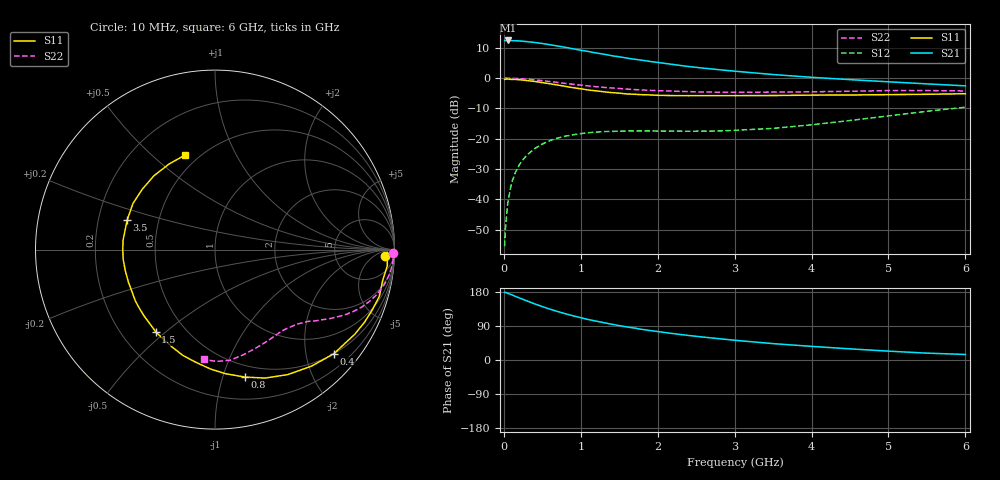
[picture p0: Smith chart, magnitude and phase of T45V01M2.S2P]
! Infineon Technologies  Discrete & RF Semiconductors
! BFR182T
! Si NPN RF Bipolar Junction Transistor in SC75
! VCE = 5 V  IC = 1.2 mA
! Common Emitter S-Parameters:  October  1999
# GHz  S  MA  R  50
!  f  S11  S21  S12  S22
! GHz  MAG  ANG  MAG  ANG  MAG  ANG  MAG  ANG
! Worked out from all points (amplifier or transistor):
!   36 points, 10 MHz to 6 GHz, reference 50 ohm
!   highest |S21| = 12.4 dB at 50 MHz (marker M1)
!   |S21| within 3 dB of that: start of sweep to 950.9 MHz
!   unconditionally stable (mu >= 1): 2.324 GHz to 4.534 GHz
!   at 250 MHz: K = 0.11, MSG = 19.5 dB, |S12| = -26.9 dB
!   at 1.4 GHz: K = 0.62, MSG = 12.5 dB, |S12| = -17.6 dB
!   at 6 GHz: K = 0.83, MSG = 3.5 dB, |S12| = -9.6 dB
!   S11 on the Smith chart (normalised r, x): 10 MHz: 25, -19; 400 MHz: 0.50, -2.58; 800 MHz: 0.39, -1.19; 1.5 GHz: 0.34, -0.46; 3.5 GHz: 0.33, +0.15; 6 GHz: 0.42, +0.64
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0.01  0.9503 -2.2  4.144 178.6  0.0017 80.0  0.9902 -1.1
0.02  0.96 -0.8  4.134 178.7  0.0032 92.0  0.9999 -0.9
0.05  0.9644 -5.4  4.171 176.0  0.0086 89.7  0.9971 -2.1
0.1  0.9502 -10.2  4.132 172.3  0.0187 84.9  0.9928 -4.2
0.15  0.9517 -16.0  4.131 168.0  0.0278 80.9  0.9876 -6.2
0.25  0.9262 -25.9  4.048 160.0  0.0454 74.3  0.9713 -10.1
0.4  0.8805 -41.2  3.867 148.1  0.0688 66.4  0.9352 -15.6
0.5  0.843 -50.4  3.713 141.0  0.0819 61.9  0.9069 -18.6
0.6  0.8058 -59.8  3.546 134.1  0.0933 57.2  0.8768 -21.5
0.7  0.7682 -68.7  3.379 127.9  0.1029 53.2  0.8466 -23.9
0.8  0.73 -76.7  3.217 122.1  0.1105 49.4  0.8174 -26.1
0.9  0.6941 -85.1  3.039 116.6  0.1163 46.5  0.7898 -28.0
1.1  0.6361 -99.9  2.742 106.7  0.126 41.1  0.7425 -31.3
1.3  0.5946 -113.3  2.478 98.5  0.1316 37.8  0.703 -34.0
1.5  0.5648 -125.8  2.244 90.8  0.1334 35.2  0.6739 -36.2
1.8  0.533 -142.6  1.968 80.7  0.1348 33.1  0.6363 -39.7
2.2  0.5152 -159.7  1.676 69.7  0.1343 33.7  0.6094 -44.0
2.8  0.5137 180.0  1.375 56.2  0.1347 38.9  0.5858 -51.7
3.5  0.5163 161.6  1.145 43.2  0.1484 48.6  0.5876 -60.7
4.5  0.5266 140.4  0.943 29.4  0.2001 58.5  0.607 -74.9
5.5  0.5411 118.3  0.803 18.1  0.2836 59.4  0.6232 -89.3
6  0.5524 107.7  0.745 14.6  0.3317 57.0  0.6146 -95.9
